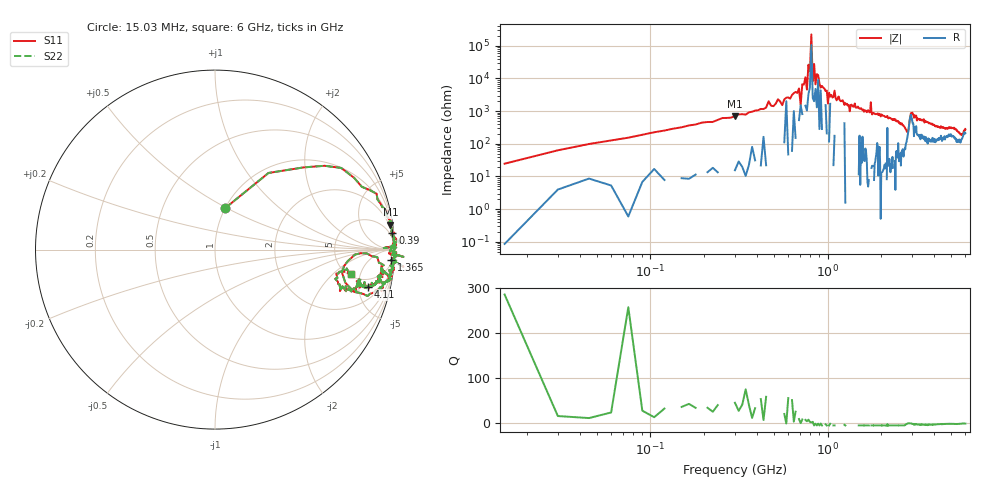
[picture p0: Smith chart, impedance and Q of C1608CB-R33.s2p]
!	Network	Analyzer	HP8753E.07.74:	Oct	30	2002	Serial	No.	JP38451487
!	Hewlett-Packard
!	28	Aug	2009	8:44:22
!	Frequency	S11	S21	S12	S22
#	HZ	S	RI	R	50
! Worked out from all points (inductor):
!   400 points, 15.03 MHz to 6 GHz, reference 50 ohm
!   read as one part in series: L = 331 nH near 45.03 MHz
!   highest Q = 40.4 at 300 MHz (marker M1), where L = 374 nH
!   self-resonance near 570 MHz
!   S11 on the Smith chart (normalised r, x): 15.03 MHz: 1.00, +0.49; 390 MHz: 2, +21; 1.365 GHz: 8, -31; 4.11 GHz: 3.52, -6.44; 6 GHz: 5.27, -3.51
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1.502992e7  0.058 0.232  0.942 -0.232  0.942 -0.232  0.058 0.232
9.002955e7  0.775 0.4  0.225 -0.4  0.225 -0.4  0.775 0.4
3.000285e8  0.977 0.138  0.0226 -0.138  0.0226 -0.138  0.977 0.138
3.90028e8  0.988 0.0949  0.012 -0.0949  0.012 -0.0949  0.988 0.0949
6.900266e8  0.997 0.0201  0.00259 -0.0201  0.00259 -0.0201  0.997 0.0201
7.050265e8  0.94 0.00897  0.0604 -0.00897  0.0604 -0.00897  0.94 0.00897
7.200264e8  0.998 0.0148  0.00204 -0.0148  0.00204 -0.0148  0.998 0.0148
7.650262e8  0.995 0.0211  0.0054 -0.0211  0.0054 -0.0211  0.995 0.0211
7.95026e8  0.998 0.00574  0.00201 -0.00574  0.00201 -0.00574  0.998 0.00574
8.10026e8  1 0.000396  0.000214 -0.000396  0.000214 -0.000396  1 0.000396
8.250259e8  0.996 0.0115  0.00388 -0.0115  0.00388 -0.0115  0.996 0.0115
8.400258e8  1 -0.0036  0.000275 0.0036  0.000275 0.0036  1 -0.0036
8.550257e8  0.989 -0.0102  0.0109 0.0102  0.0109 0.0102  0.989 -0.0102
1.020025e9  0.998 -0.0272  0.00162 0.0272  0.00162 0.0272  0.998 -0.0272
1.365023e9  0.982 -0.0598  0.0181 0.0598  0.0181 0.0598  0.982 -0.0598
2.01002e9  0.982 -0.124  0.0177 0.124  0.0177 0.124  0.982 -0.124
2.820016e9  0.726 -0.184  0.274 0.184  0.274 0.184  0.726 -0.184
3.015015e9  0.94 -0.0869  0.0597 0.0869  0.0597 0.0869  0.94 -0.0869
4.00501e9  0.872 -0.209  0.128 0.209  0.128 0.209  0.872 -0.209
4.110009e9  0.854 -0.208  0.146 0.208  0.146 0.208  0.854 -0.208
5.010005e9  0.805 -0.179  0.195 0.179  0.195 0.179  0.805 -0.179
6e9  0.757 -0.136  0.243 0.136  0.243 0.136  0.757 -0.136
